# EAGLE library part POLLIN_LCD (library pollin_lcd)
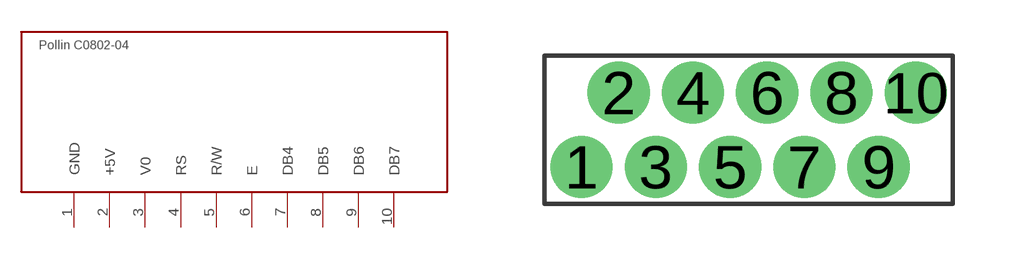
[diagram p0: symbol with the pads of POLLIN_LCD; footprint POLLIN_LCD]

Designator prefix -

## POLLIN_LCD  [POLLIN_LCD]
1  GND
2  +5V
3  V0
4  RS
5  R/W
6  E
7  DB4
8  DB5
9  DB6
10  DB7

## Footprint POLLIN_LCD (pad centres in mm)
drill 0.5 pad 1.676: 1 -5,-1; 2 -4,1; 3 -3,-1; 4 -2,1; 5 -1,-1; 6 0,1; 7 1,-1; 8 2,1; 9 3,-1; 10 4,1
